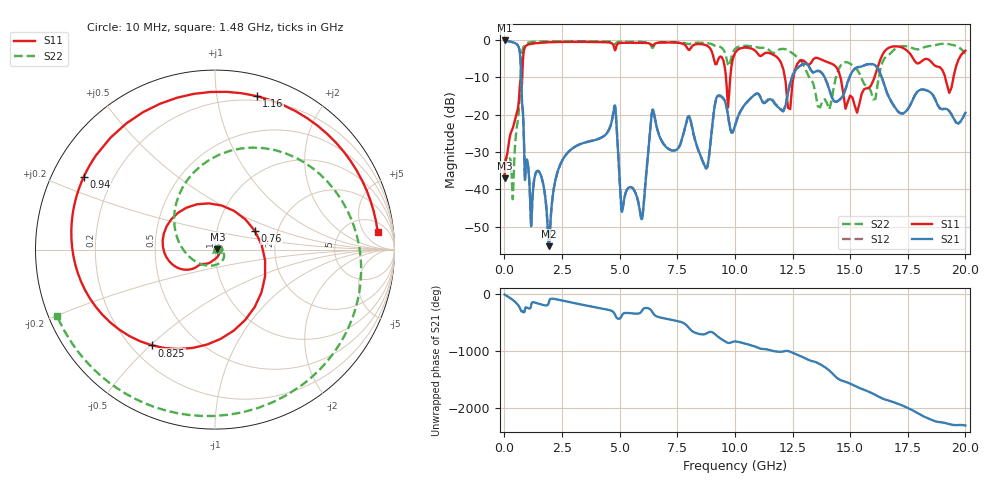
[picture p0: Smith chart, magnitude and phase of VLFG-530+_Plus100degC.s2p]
! Mini-Circuits
! S2P DATA File Format
! Type: LOW PASS FILTER
! Model: VLFG-530+
! All S Parameters are in dB deg format
! TEST CONDITIONS: INPUT POWER = 0 dBm @ Temperature = +100 deg C
# MHz S dB R 50
!Frequency  S11 dB  S11 DEG  S21 dB  S21 DEG  S12 dB  S12 DEG  S22 dB  S22 DEG
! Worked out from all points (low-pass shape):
!   652 points, 10 MHz to 20 GHz, reference 50 ohm
!   highest |S21| = -0.13 dB at 10 MHz (marker M1); lowest = -55.2 dB at 1.94 GHz (marker M2)
!   |S21| within 3 dB of the highest: start of sweep to 665.1 MHz
!   lowest |S11| = -37.0 dB at 11 MHz (marker M3), VSWR 1.03, Z = 51.4 + j0.284 ohm
!   |S11| at or under -10 dB: start of sweep to 774.9 MHz; 12.17 GHz to 12.54 GHz (376 MHz wide, 3.04 % of centre); 14.58 GHz to 16.05 GHz (1.475 GHz wide, 9.63 % of centre)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
!   |S22| runs from -42.6 to -0.3 dB; largest |S21 - S12| = 0.012
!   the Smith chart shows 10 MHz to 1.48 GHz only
!   S11 on the Smith chart (normalised r, x): 10 MHz: 1.03, +0.00; 760 MHz: 1.53, +0.33; 825 MHz: 0.28, -0.51; 940 MHz: 0.10, +0.26; 1.16 GHz: 0.16, +1.29; 1.48 GHz: 9, +11
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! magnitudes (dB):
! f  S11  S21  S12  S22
! 10 MHz  -37.0  -0.1  -0.1  -36.8
! 11 MHz  -37.0  -0.1  -0.1  -36.9
! 365 MHz  -23.5  -0.6  -0.6  -42.6
! 760 MHz  -12.2  -16.0  -16.0  -3.6
! 825 MHz  -3.9  -22.0  -22.0  -1.9
! 940 MHz  -1.6  -32.8  -32.8  -1.0
! 1.16 GHz  -1.0  -49.9  -49.9  -0.6
! 1.48 GHz  -0.8  -35.1  -35.1  -0.4
! 1.94 GHz  -0.6  -55.2  -55.2  -0.3
! 2.36 GHz  -0.5  -34.4  -34.4  -0.3
! 3.35 GHz  -0.5  -27.7  -27.7  -0.3
! 4.775 GHz  -2.3  -17.7  -17.6  -1.0
! 5.1 GHz  -0.8  -46.0  -46.0  -0.4
! 5.95 GHz  -0.8  -48.0  -47.9  -0.5
! 6.4 GHz  -1.4  -19.5  -19.4  -2.0
! 6.675 GHz  -0.8  -24.8  -24.7  -0.7
! 8.7 GHz  -1.3  -33.9  -34.1  -0.8
! 10.05 GHz  -3.1  -22.0  -22.1  -2.2
! 13.4 GHz  -5.2  -8.7  -8.8  -11.6
! 15.1 GHz  -15.4  -8.4  -8.4  -6.8
! 16.7 GHz  -2.0  -15.5  -15.7  -3.9
! 20 GHz  -2.9  -19.5  -19.5  -3.9
